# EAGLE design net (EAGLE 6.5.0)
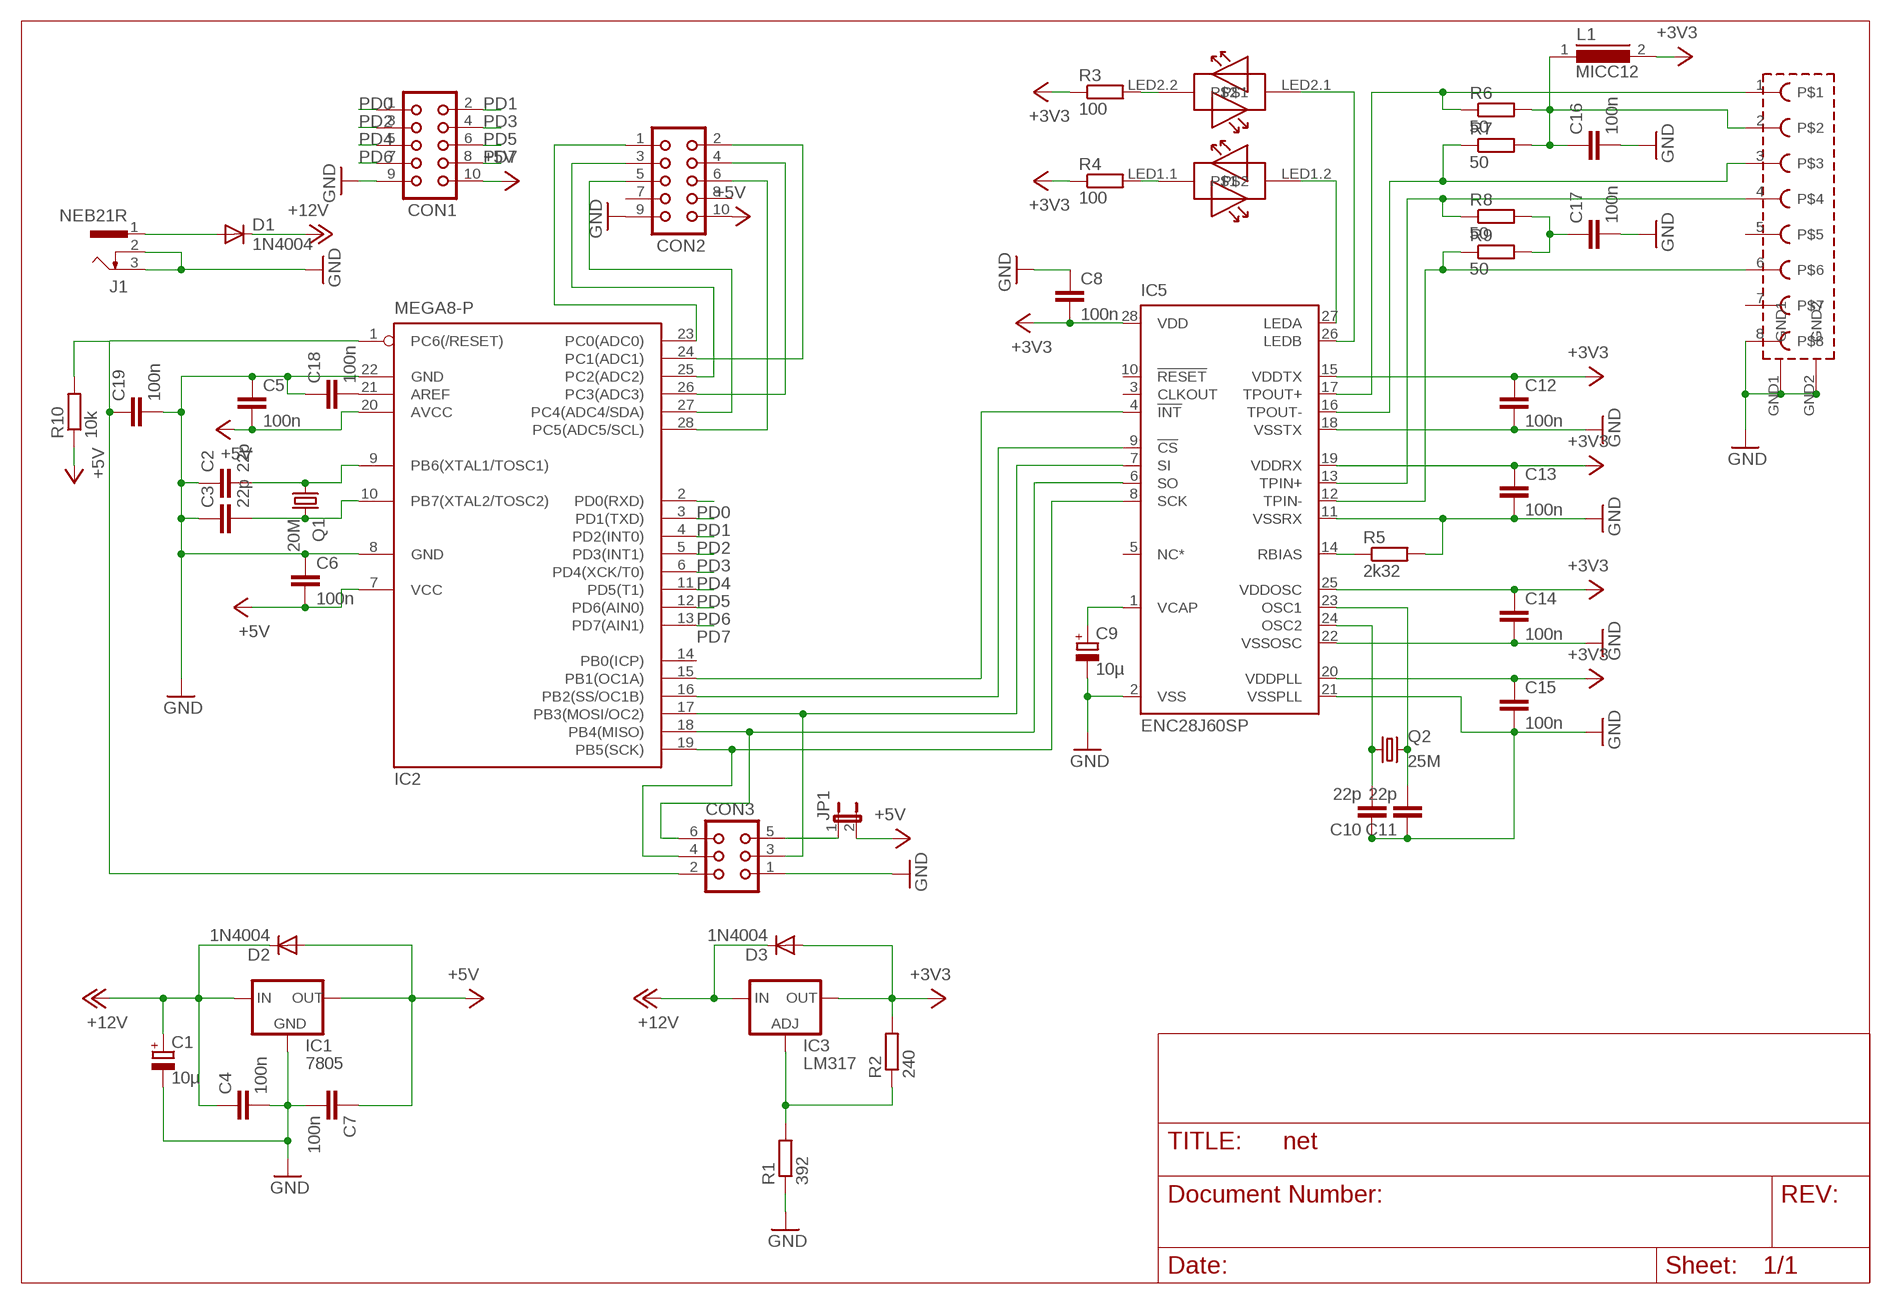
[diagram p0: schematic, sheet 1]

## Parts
C1  10µ  CPOL-EUE2.5-5  [E2,5-5]
C2  22p  C-EU025-025X050  [C025-025X050]
C3  22p  C-EU025-025X050  [C025-025X050]
C4  100n  C-EU025-025X050  [C025-025X050]
C5  100n  C-EU025-025X050  [C025-025X050]
C6  100n  C-EU025-025X050  [C025-025X050]
C7  100n  C-EU025-025X050  [C025-025X050]
C8  100n  C-EU025-025X050  [C025-025X050]
C9  10µ  CPOL-EUE2-4  [E2-4]
C10  22p  C-EU025-025X050  [C025-025X050]
C11  22p  C-EU025-025X050  [C025-025X050]
C12  100n  C-EU025-025X050  [C025-025X050]
C13  100n  C-EU025-025X050  [C025-025X050]
C14  100n  C-EU025-025X050  [C025-025X050]
C15  100n  C-EU025-025X050  [C025-025X050]
C16  100n  C-EU025-025X050  [C025-025X050]
C17  100n  C-EU025-025X050  [C025-025X050]
C18  100n  C-EU025-025X050  [C025-025X050]
C19  100n  C-EU025-025X050  [C025-025X050]
CON1  CON10  [CON10]
CON2  CON10  [CON10]
CON3  CON06  [CON06]
D1  1N4004  [DO41-10]
D2  1N4004  [DO41-10]
D3  1N4004  [DO41-10]
IC1  7805  78XXS  [78XXS]
IC2  MEGA8-P  [DIL28-3]
IC3  LM317  LM317TS  [317TS]
IC5  ENC28J60SP  [DIL28-3]
J1  NEB21R  [NEB21R]
JP1  JP1E  [JP1]
L1  MICC12  [MICC12]
Q1  20M  CRYSTALHC49U-V  [HC49U-V]
Q2  25M  CRYSTALHC49U-V  [HC49U-V]
R1  392  R-EU_0207/10  [0207/10]
R2  240  R-EU_0207/10  [0207/10]
R3  100  R-EU_0207/10  [0207/10]
R4  100  R-EU_0207/10  [0207/10]
R5  2k32  R-EU_0207/10  [0207/10]
R6  50  R-EU_0207/10  [0207/10]
R7  50  R-EU_0207/10  [0207/10]
R8  50  R-EU_0207/10  [0207/10]
R9  50  R-EU_0207/10  [0207/10]
R10  10k  R-EU_0207/10  [0207/10]
U$1  MAGJACK  [MAGJACK]

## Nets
+3V3: C8.2 C12.1 C13.1 C14.1 C15.1 D3.A IC3.2(OUT) IC5.15(VDDTX) IC5.19(VDDRX) IC5.20(VDDPLL) IC5.25(VDDOSC) IC5.28(VDD) L1.2 R2.2 R3.1 R4.1
+5V: C5.2 C6.2 C7.1 CON1.10 CON2.10 D2.A IC1.OUT IC2.7(VCC) IC2.20(AVCC) JP1.2 R10.1
+12V: C1.+ C4.1 D1.C D2.C D3.C IC1.IN IC3.3(IN)
GND: C1.- C2.1 C3.1 C4.2 C5.1 C6.1 C7.2 C8.1 C9.- C10.1 C11.1 C12.2 C13.2 C14.2 C15.2 C16.2 C17.2 C18.1 C19.2 CON1.9 CON2.9 CON3.1 IC1.GND IC2.8(GND) IC2.22(GND) IC5.2(VSS) IC5.11(VSSRX) IC5.18(VSSTX) IC5.21(VSSPLL) IC5.22(VSSOSC) J1.2 J1.3 R1.1 R5.2 U$1.8 U$1.GND1 U$1.GND2
N$1: CON3.5 JP1.1
N$2: CON3.6 IC2.18(PB4(MISO)) IC5.6(SO)
N$3: IC2.16(PB2(SS/OC1B)) IC5.9(!CS)
N$4: IC2.15(PB1(OC1A)) IC5.4(!INT)
N$5: C2.2 IC2.9(PB6(XTAL1/TOSC1)) Q1.1
N$6: C3.2 IC2.10(PB7(XTAL2/TOSC2)) Q1.2
N$7: C9.+ IC5.1(VCAP)
N$8: IC5.14(RBIAS) R5.1
N$10: IC5.17(TPOUT+) R6.1 U$1.1
N$11: R4.2 U$1.LED1.1
N$12: CON3.3 IC2.17(PB3(MOSI/OC2)) IC5.7(SI)
N$13: IC5.16(TPOUT-) R7.1 U$1.3
N$14: C18.2 IC2.21(AREF)
N$15: IC5.13(TPIN+) R8.1 U$1.4
N$16: C10.2 IC5.24(OSC2) Q2.1
N$17: C11.2 IC5.23(OSC1) Q2.2
N$18: IC5.12(TPIN-) R9.1 U$1.6
N$19: C16.1 L1.1 R6.2 R7.2 U$1.2
N$20: C17.1 R8.2 R9.2
N$21: D1.A J1.1
N$23: R3.2 U$1.LED2.2
N$24: IC5.27(LEDA) U$1.LED1.2
N$25: IC5.26(LEDB) U$1.LED2.1
N$26: CON2.1 IC2.23(PC0(ADC0))
N$27: IC3.1(ADJ) R1.2 R2.1
N$28: CON2.2 IC2.24(PC1(ADC1))
N$29: CON2.3 IC2.25(PC2(ADC2))
N$30: CON2.5 IC2.27(PC4(ADC4/SDA))
N$31: CON2.4 IC2.26(PC3(ADC3))
N$32: CON2.6 IC2.28(PC5(ADC5/SCL))
N$34: CON3.4 IC2.19(PB5(SCK)) IC5.8(SCK)
N$37: C19.1 CON3.2 IC2.1(PC6(/RESET)) R10.2
PD0: CON1.1 IC2.2(PD0(RXD))
PD1: CON1.2 IC2.3(PD1(TXD))
PD2: CON1.3 IC2.4(PD2(INT0))
PD3: CON1.4 IC2.5(PD3(INT1))
PD4: CON1.5 IC2.6(PD4(XCK/T0))
PD5: CON1.6 IC2.11(PD5(T1))
PD6: CON1.7 IC2.12(PD6(AIN0))
PD7: CON1.8 IC2.13(PD7(AIN1))
Unconnected: CON2.7 CON2.8 IC2.14(PB0(ICP)) IC5.3(CLKOUT) IC5.5(NC*) IC5.10(!RESET) U$1.5 U$1.7

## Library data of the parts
C1 C9 = rcl:CPOL-EU: POLARIZED CAPACITOR, European symbol
C2 C3 C5 C6 C8 C10-C19 = resistor:C-EU: CAPACITOR, European symbol
C4 C7 = rcl:C-EU: CAPACITOR, European symbol
CON1 CON2 = con-harting:CON10: CONNECTOR; OC_FARNELL: unknown; OC_NEWARK: unknown
CON3 = con-harting:CON06: CONNECTOR; OC_FARNELL: unknown; OC_NEWARK: unknown
D1-D3 = diode:1N4004: DIODE
IC1 = v-reg:78XXS: VOLTAGE REGULATOR
IC2 = atmel:MEGA8-P: MICROCONTROLLER 8 Kbytes FLASH, 1 kbytes SRAM, 512 bytes EEPROM, USART, 4-channel 10 bit ADC, 2-channel 8 bit ADC Pin compatible with Atmega48, ATMega88, ATMega168 Source: avr.lbr; OC_FARNELL: unknown; OC_NEWARK: unknown
IC3 = v-reg:LM317TS: VOLTAGE REGULATOR
IC5 = microchip:ENC28J60: Stand-Alone Ethernet Controller with SPI Interface Source: http://ww1.microchip.com/downloads/en/DeviceDoc/39662c.pdf; MF: MICROCHIP; MPN: ENC28J60/SP; OC_FARNELL: 1084619; OC_NEWARK: 96K3661
J1 = con-lumberg:NEB21R: Netzgeräte-Einbaukupplung abgewinkelte Ausführung mit Öffner Source: http://www.lumberg.com/Produkte/PDFs/NEB21R.pdf; MPN: NEB 21 R; OC_FARNELL: 1217037; OC_NEWARK: 97K6458
JP1 = jumper:JP1E: JUMPER
L1 = inductors:MICC12: INDUCTOR
Q1 Q2 = crystal:CRYSTAL: CRYSTAL; OC_FARNELL: 1666969; OC_NEWARK: unknown
R1-R10 = rcl:R-EU_: RESISTOR, European symbol
U$1 = magjacksmalldrill:MAGJACK

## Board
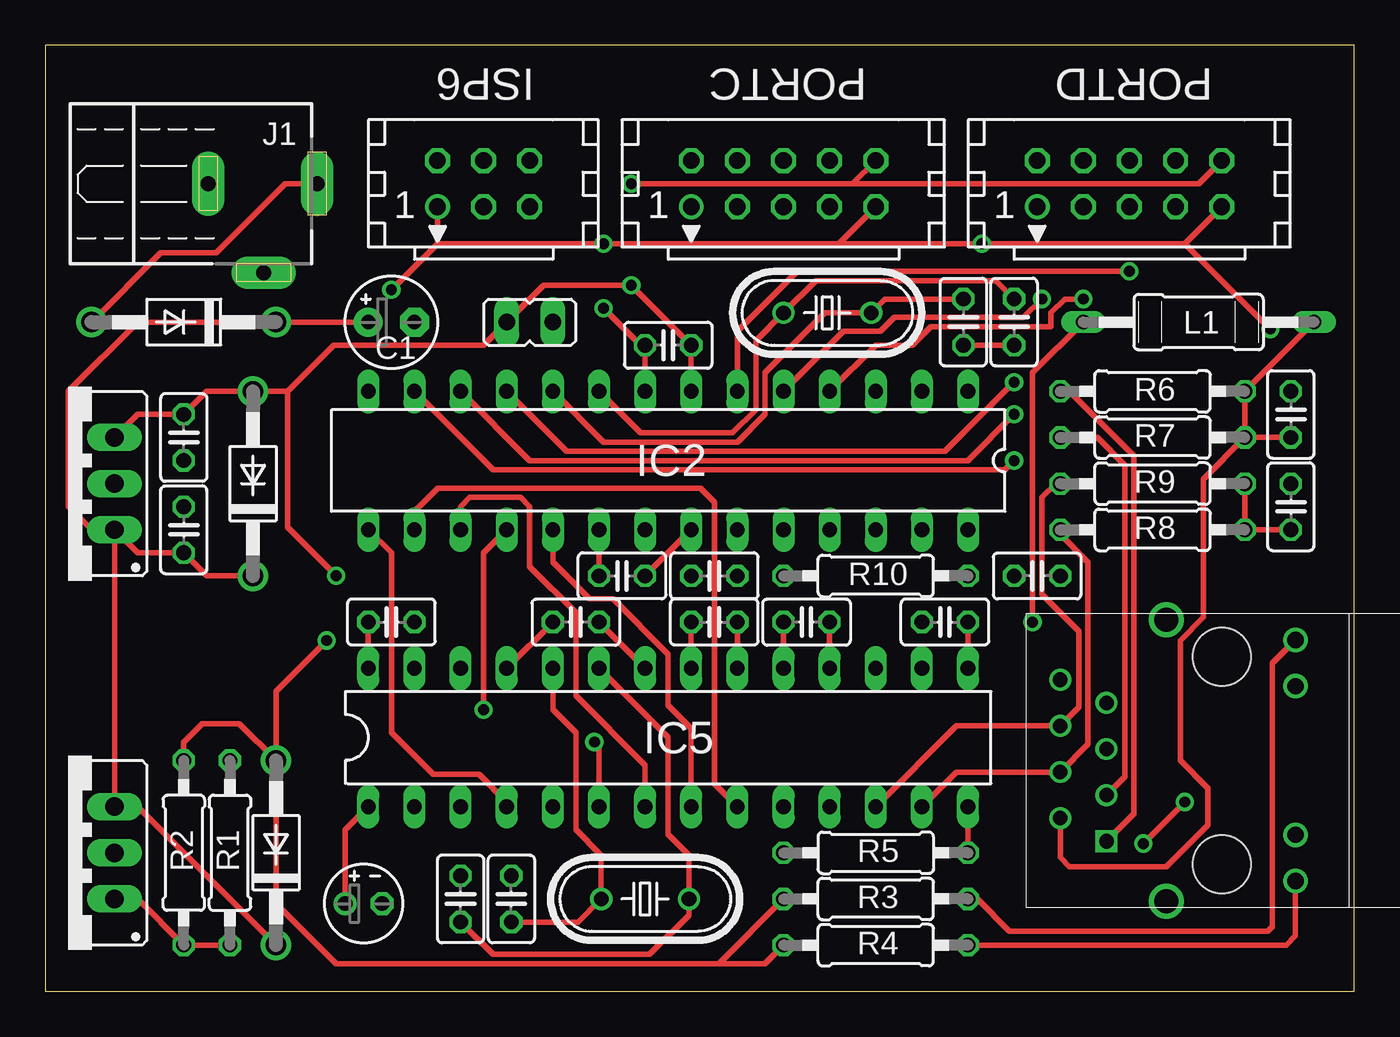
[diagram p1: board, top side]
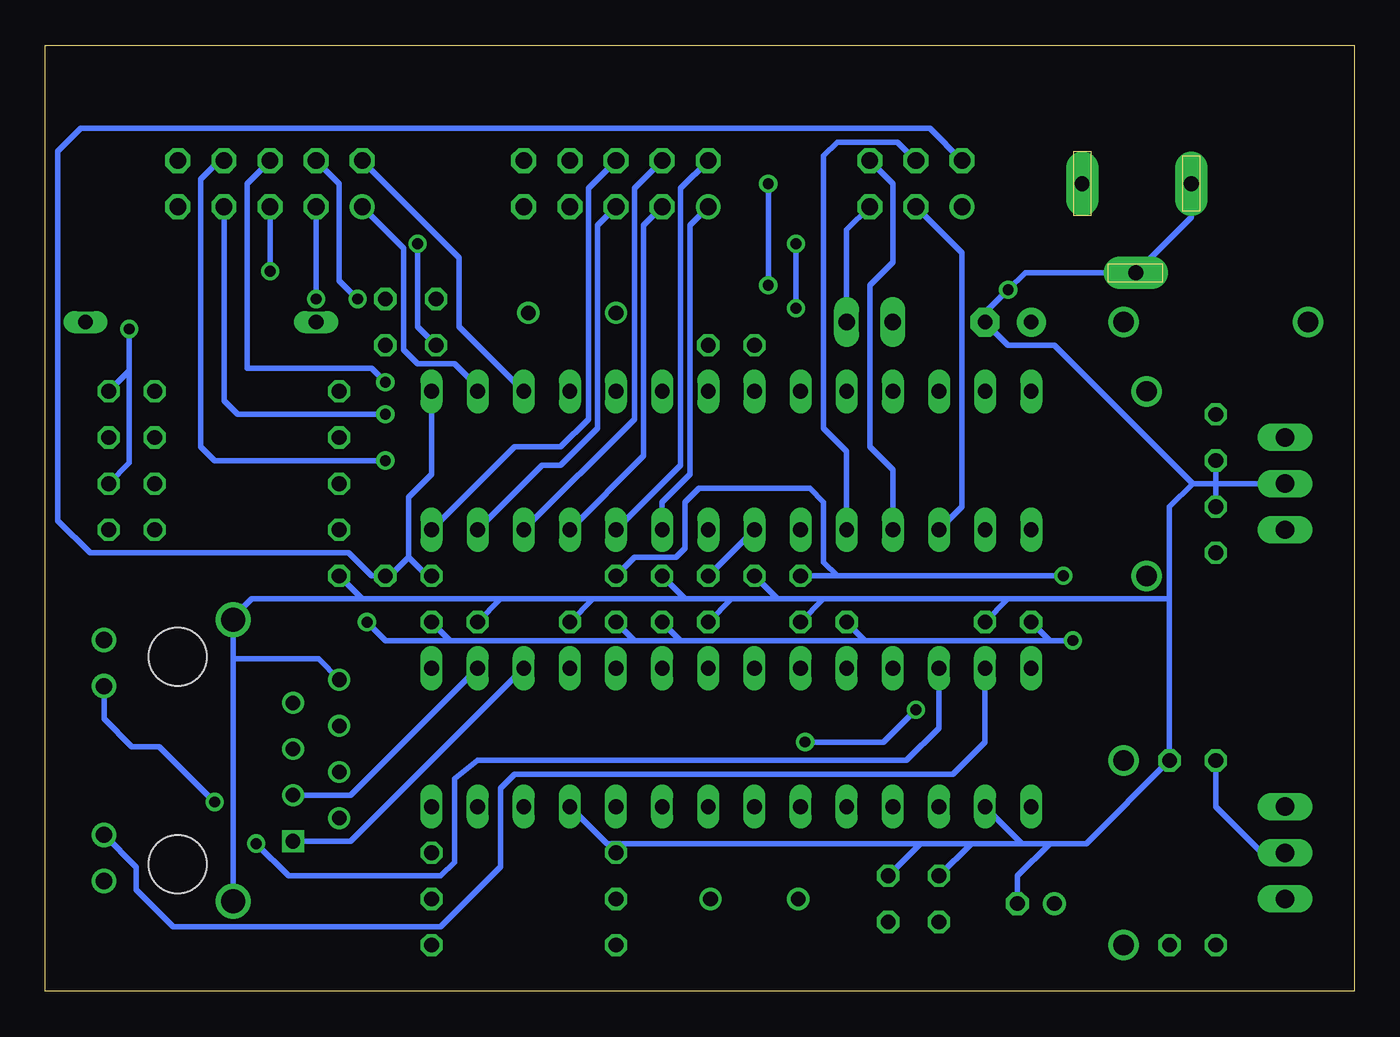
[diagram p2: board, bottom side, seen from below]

Size 72.06 x 52.06 mm. Coordinates in mm from the lower left corner, seen from the top.
Outline: 0,0 72.06,0 72.06,52.06 0,52.06 0,0
Copper layers (1*16): Top 0.035mm / dielectric 1.5mm / Bottom 0.035mm
Design rules "platinensammler_02": minimum track width 0.15mm, minimum drill 0.3mm, track to track 0.15mm, track to pad 0.15mm, pad to pad 0.15mm, via to via 0.15mm, smd to smd 0mil, copper to edge 0.2mm, drill to drill 0.2mm, minimum pad ring 0.2mm, minimum via ring 0.2mm, stop-mask expansion 4mil, vias tented up to drill 0.8mm, thermal gap 0.15mm

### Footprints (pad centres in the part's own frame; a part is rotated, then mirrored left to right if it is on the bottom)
E2,5-5 = drill 0.813 pad 1.6: + -1.27,0 | drill 0.813 pad 1.6 octagon: - 1.27,0
C025-025X050 = drill 0.813 octagon: 1 -1.27,0; 2 1.27,0
E2-4 = drill 0.813 pad 1.27: + -1.016,0 | drill 0.813 pad 1.27 octagon: - 1.016,0
CON10 = drill 0.914: 1 -5.08,-1.27 | drill 0.914 octagon: 2 -5.08,1.27; 3 -2.54,-1.27; 4 -2.54,1.27; 5 0,-1.27; 6 0,1.27; 7 2.54,-1.27; 8 2.54,1.27; 9 5.08,-1.27; 10 5.08,1.27
CON06 = drill 0.914: 1 -2.54,-1.27 | drill 0.914 octagon: 2 -2.54,1.27; 3 0,-1.27; 4 0,1.27; 5 2.54,-1.27; 6 2.54,1.27
DO41-10 = drill 1.118: A 5.08,0; C -5.08,0
78XXS = drill 1.016 long: GND 0,-2.54; IN -2.54,-2.54; OUT 2.54,-2.54
DIL28-3 = drill 0.813 long: 1 -16.51,-3.81; 2 -13.97,-3.81; 3 -11.43,-3.81; 4 -8.89,-3.81; 5 -6.35,-3.81; 6 -3.81,-3.81; 7 -1.27,-3.81; 8 1.27,-3.81; 9 3.81,-3.81; 10 6.35,-3.81; 11 8.89,-3.81; 12 11.43,-3.81; 13 13.97,-3.81; 14 16.51,-3.81; 15 16.51,3.81; 16 13.97,3.81; 17 11.43,3.81; 18 8.89,3.81; 19 6.35,3.81; 20 3.81,3.81; 21 1.27,3.81; 22 -1.27,3.81; 23 -3.81,3.81; 24 -6.35,3.81; 25 -8.89,3.81; 26 -11.43,3.81; 27 -13.97,3.81; 28 -16.51,3.81
317TS = drill 1.016 long: 1 -2.54,-2.54; 2 0,-2.54; 3 2.54,-2.54
NEB21R = drill 0.813 pad 1.778 long: 1 0,7.35; 2 4.9,4.4; 3 0,1.35
JP1 = drill 0.914 long: 1 0,-1.27; 2 0,1.27
MICC12 = drill 0.813 long: 1 -6.35,0; 2 6.35,0
HC49U-V = drill 0.813: 1 -2.413,0; 2 2.413,0
0207/10 = drill 0.813 octagon: 1 -5.08,0; 2 5.08,0
MAGJACK = drill 0.8 square: 1 -4.445,6.35 | drill 0.8: 2 -3.175,8.89; 3 -1.905,6.35; 4 -0.635,8.89; 5 0.635,6.35; 6 1.905,8.89; 7 3.175,6.35; 8 4.445,8.89 | drill 1.3: GND1 -7.747,3.048; GND2 7.747,3.048 | drill 0.9: LED1.1 -6.629,-4.064; LED1.2 -4.089,-4.064; LED2.1 4.089,-4.064; LED2.2 6.629,-4.064 | hole 3.2: -5.715,0; 5.715,0

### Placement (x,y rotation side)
C1  19.05,36.83 0 top
C2  53.34,36.83 90 top
C3  50.55,36.83 90 top
C4  7.62,25.4 90 top
C5  34.29,35.56 0 top
C6  31.75,22.86 180 top
C7  7.62,30.48 270 top
C8  19.05,20.32 180 top
C9  17.53,4.83 0 top
C10  25.65,5.08 270 top
C11  22.86,5.08 270 top
C12  41.91,20.32 0 top
C13  49.53,20.32 180 top
C14  29.21,20.32 0 top
C15  36.83,20.32 180 top
C16  68.58,31.75 90 top
C17  68.58,26.67 90 top
C18  36.83,22.86 180 top
C19  54.61,22.86 0 top
CON1  59.69,44.45 0 top
CON2  40.64,44.45 0 top
CON3  24.13,44.45 0 top
D1  7.62,36.83 180 top
D2  11.43,27.94 90 top
D3  12.7,7.62 90 top
IC1  1.27,27.94 90 top
IC2  34.29,29.21 180 top
IC3  1.27,7.62 90 top
IC5  34.29,13.97 0 top
J1  7.62,44.45 270 top
JP1  26.67,36.83 90 top
L1  63.5,36.83 180 top
Q1  43.05,37.34 0 top
Q2  33.02,5.08 0 top
R1  10.16,7.62 270 top
R2  7.62,7.62 90 top
R3  45.72,5.08 0 top
R4  45.72,2.54 0 top
R5  45.72,7.62 180 top
R6  60.96,33.02 0 top
R7  60.96,30.48 0 top
R8  60.96,25.4 0 top
R9  60.96,27.94 0 top
R10  45.72,22.86 0 top
U$1  64.77,12.7 90 top

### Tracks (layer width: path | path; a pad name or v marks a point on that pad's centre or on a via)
+3V3  (via drill 0.6)
  Top 0.305: C15.1 IC5.20 | C12.1 IC5.19 | C13.1 IC5.15 | R2.2 7.62,13.72 8.64,14.73 10.67,14.73 D3.A | L1.2 54.36,34.04 v54.36,20.32 | R4.1 39.62,1.52 37.08,1.52 | 37.08,1.52 16,1.52 12.7,4.83 D3.A | R3.1 37.08,1.52 | D3.A 12.7,16.51 v15.49,19.3 | IC5.28 C8.2 | C14.1 IC5.25
  Bottom 0.305: IC3.2 5.08,7.62 7.62,10.16 R2.2 | v15.49,19.3 16.76,19.3 | 16.76,19.3 26.92,19.3 | 26.92,19.3 37.08,19.3 | 37.08,19.3 39.62,19.3 | 39.62,19.3 49.78,19.3 | 49.78,19.3 53.34,19.3 v54.36,20.32 | C8.2 16.76,19.3 | C15.1 37.08,19.3 | C12.1 39.62,19.3 | C13.1 49.78,19.3 | C14.1 26.92,19.3
+5V  (via drill 0.6)
  Top 0.305: IC2.7 C5.2 v32.26,38.86 27.43,38.86 JP1.2 24.13,35.56 15.88,35.56 13.34,33.02 | IC1.OUT 5.08,31.75 C7.1 8.89,33.02 D2.A 13.34,33.02 | 13.34,33.02 13.34,25.53 v16,22.86 | CON1.10 63.5,44.45 44.45,44.45 | 44.45,44.45 v32.26,44.45 | CON2.10 44.45,44.45 | IC2.20 C6.2
  Bottom 0.305: v16,22.86 26.92,22.86 28.45,22.86 | 28.45,22.86 C6.2 | v32.26,44.45 v32.26,38.86 | R10.1 39.62,23.88 37.34,23.88 36.83,24.38 36.83,26.92 36.07,27.69 29.97,27.69 29.21,26.92 29.21,23.62 28.45,22.86
+12V
  Top 0.305: IC1.IN 2.54,25.4 1.27,26.67 1.27,33.02 5.08,36.83 D1.C C1.+ | IC1.IN 5.08,24.13 C4.1 8.89,22.86 D2.C | IC1.IN IC3.3 5.08,10.16 D3.C
GND  (via drill 0.6)
  Top 0.305: IC5.21 C15.2 | IC5.18 C12.2 | C5.1 IC2.8 33.02,35.31 v30.73,37.59 | IC5.22 C14.2 | CON3.1 21.59,41.15 | 21.59,41.15 v19.05,38.61 | CON2.9 43.69,41.15 | 43.69,41.15 v30.73,41.15 21.59,41.15 | CON1.9 62.74,41.15 | 62.74,41.15 v51.56,41.15 43.69,41.15 | C3.1 C2.1 | 62.74,41.15 v67.44,36.45 | IC2.22 C6.1
  Bottom 0.305: IC1.GND 7.62,27.94 | C7.2 7.62,27.94 | C4.2 7.62,27.94 | U$1.GND1 61.72,18.29 | 61.72,18.29 U$1.GND2 61.72,20.57 60.71,21.59 54.61,21.59 | U$1.8 57.02,18.29 61.72,18.29 | 18.29,8.13 16.76,8.13 | 16.76,8.13 14.73,8.13 R1.1 10.16,21.59 | C11.1 21.08,8.13 | 21.08,8.13 18.29,8.13 | C10.1 23.88,8.13 | 23.88,8.13 21.08,8.13 | R5.2 40.13,8.13 | 40.13,8.13 23.88,8.13 | IC5.2 18.29,8.13 | IC5.11 41.15,8.13 40.13,8.13 | 7.62,27.94 8.89,27.94 | 8.89,27.94 10.16,26.67 10.16,21.59 | C13.2 46.99,21.59 | 46.99,21.59 41.91,21.59 | 41.91,21.59 36.83,21.59 | 34.29,21.59 31.75,21.59 | 29.21,21.59 19.05,21.59 | 19.05,21.59 10.16,21.59 | C8.1 19.05,21.59 | C15.2 34.29,21.59 | C12.2 41.91,21.59 | C16.2 67.44,34.16 | C17.2 67.44,29.08 67.44,34.16 | 54.61,21.59 46.99,21.59 | 67.44,34.16 v67.44,36.45 | 8.89,27.94 16.51,35.56 19.05,35.56 C1.- 20.32,37.34 v19.05,38.61 18.11,39.55 J1.2 8.97,42.6 J1.3 | v30.73,37.59 v30.73,41.15 | C3.1 51.56,36.58 v51.56,41.15 | C14.2 29.21,21.59 | C6.1 31.75,21.59 | 31.75,21.59 29.21,21.59 | C18.1 36.83,21.59 | 36.83,21.59 34.29,21.59 | C19.2 54.61,21.59 | C9.- 18.54,6.35 16.76,8.13
N$1
  Bottom 0.305: CON3.5 27.94,41.91 JP1.1
N$2  (via drill 0.6)
  Top 0.305: IC5.6 30.48,13.46 v30.23,13.72 | v24.13,15.49 24.13,24.13 IC2.18
  Bottom 0.305: v30.23,13.72 25.91,13.72 v24.13,15.49 | CON3.6 25.4,44.45 25.4,40.13 26.67,38.86 26.67,29.97 25.4,28.7 IC2.18
N$3
  Top 0.305: IC5.9 36.83,11.43 36.83,26.92 36.07,27.69 21.59,27.69 20.32,26.42 IC2.16
N$4
  Top 0.305: IC2.15 19.05,24.13 19.05,14.22 21.34,11.94 23.88,11.94 25.4,10.41 IC5.4
N$5
  Top 0.305: IC2.9 32.77,30.73 37.85,30.73 39.12,32 39.12,35.81 Q1.1 42.42,39.12 52.32,39.12 C2.2
N$6
  Top 0.305: IC2.10 30.73,30.23 38.1,30.23 39.62,31.75 39.62,34.04 42.93,37.34 Q1.2 46.23,38.1 C3.2
N$7
  Top 0.305: IC5.1 16.51,8.89 C9.+
N$8
  Top 0.305: IC5.14 R5.1
N$10
  Top 0.305: R6.1 56.39,33.02 59.94,29.46 59.94,9.78 U$1.1
  Bottom 0.305: IC5.17 55.24,8.26 U$1.1
N$11
  Top 0.305: U$1.LED1.1 68.83,3.05 68.33,2.54 R4.2
N$12
  Top 0.305: IC5.7 33.02,12.45 29.21,16.26 29.21,20.83 26.67,23.37 26.67,26.67 26.16,27.18 23.37,27.18 22.86,26.67 IC2.17
  Bottom 0.305: CON3.3 21.59,40.64 21.59,26.67 IC2.17
N$13
  Top 0.305: R7.1 57.91,30.48 59.44,28.96 59.44,11.81 U$1.3
  Bottom 0.305: IC5.16 55.24,10.79 U$1.3
N$14
  Bottom 0.305: IC2.21 C18.2
N$15
  Top 0.305: IC5.13 50.16,12.06 U$1.4 57.4,13.59 57.4,23.62 55.88,25.15 R8.1
N$16
  Top 0.305: C10.2 29.34,3.81 Q2.1 30.61,7.49 29.21,8.89 29.21,14.22 27.94,15.49 IC5.24
N$17
  Top 0.305: IC5.23 34.29,13.97 34.29,8.64 35.43,7.49 Q2.2 35.43,4.19 33.27,2.03 24.64,2.03 C11.2
N$18
  Top 0.305: IC5.12 50.16,14.61 U$1.6 56.9,15.62 56.9,19.81 54.86,21.84 54.86,27.18 55.63,27.94 R9.1
N$19
  Top 0.305: R7.2 R6.2 L1.1 | R7.2 C16.1 | R7.2 63.75,28.19 63.75,20.57 62.48,19.3 62.48,12.7 64.01,11.18 64.01,9.14 61.72,6.86 56.39,6.86 55.88,7.37 U$1.2
N$20
  Top 0.305: R9.2 R8.2 C17.1
N$21
  Top 0.305: J1.1 13.21,44.45 9.4,40.64 6.35,40.64 D1.A
N$23
  Top 0.305: U$1.LED2.2 67.56,18.06 67.56,3.56 67.31,3.3 53.09,3.3 51.31,5.08 R3.2
N$24
  Bottom 0.305: IC5.27 20.32,13.72 22.1,11.94 46.23,11.94 46.99,11.18 46.99,6.86 50.29,3.56 65.02,3.56 67.06,5.59 67.06,6.83 U$1.LED1.2
N$25  (via drill 0.6)
  Top 0.305: v60.45,8.13 v62.74,10.41
  Bottom 0.305: IC5.26 22.86,14.48 24.64,12.7 48.26,12.7 49.53,11.68 49.53,7.11 50.29,6.35 58.67,6.35 v60.45,8.13 | v62.74,10.41 65.79,13.46 67.31,13.46 68.83,14.99 U$1.LED2.1
N$26
  Bottom 0.305: CON2.1 36.58,42.16 36.58,28.45 38.1,26.92 IC2.23
N$27
  Top 0.305: IC3.1 5.08,5.08 R2.1 R1.2
N$28
  Bottom 0.305: CON2.2 37.08,44.2 37.08,28.96 IC2.24
N$29
  Bottom 0.305: CON2.3 39.12,42.16 39.12,29.46 IC2.25
N$30
  Bottom 0.305: CON2.5 41.66,42.16 41.66,30.99 43.69,28.96 44.7,28.96 IC2.27
N$31
  Bottom 0.305: CON2.4 39.62,44.2 39.62,31.5 IC2.26
N$32
  Bottom 0.305: CON2.6 42.16,44.2 42.16,31.5 43.69,29.97 46.23,29.97 IC2.28
N$34
  Top 0.305: IC5.8 35.56,14.48 34.29,15.75 34.29,18.54 31.24,21.59 29.97,21.59 27.94,23.62 IC2.19
  Bottom 0.305: CON3.4 25.15,46.74 28.45,46.74 29.21,45.97 29.21,30.99 27.94,29.72 IC2.19
N$37
  Bottom 0.305: IC2.1 50.8,28.45 52.07,27.18 52.07,23.88 | CON3.2 23.37,47.5 70.1,47.5 71.37,46.23 71.37,25.91 69.6,24.13 55.37,24.13 54.1,22.86 C19.1 53.09,22.86 52.07,23.88 | 52.07,23.88 51.05,22.86 R10.2
PD0
  Bottom 0.305: IC2.2 48.26,33.27 49.53,34.54 51.56,34.54 52.32,35.31 52.32,40.89 CON1.1
PD1
  Bottom 0.305: IC2.3 49.28,36.58 49.28,40.39 CON1.2
PD2  (via drill 0.6)
  Top 0.305: IC2.4 45.72,35.56 47.75,35.56 48.77,36.58 55.37,36.58 55.37,37.34 56.13,38.1 v57.15,38.1
  Bottom 0.305: v57.15,38.1 CON1.3
PD3  (via drill 0.6)
  Top 0.305: IC2.5 43.94,36.32 45.97,36.32 46.74,37.08 53.85,37.08 v54.86,38.1
  Bottom 0.305: CON1.4 55.88,44.45 55.88,39.12 v54.86,38.1
PD4  (via drill 0.6)
  Top 0.305: IC2.6 38.1,36.32 41.4,39.62 v59.69,39.62
  Bottom 0.305: v59.69,39.62 CON1.5
PD5  (via drill 0.6)
  Top 0.305: IC2.11 28.7,29.72 49.53,29.72 v53.34,33.53
  Bottom 0.305: v53.34,33.53 54.1,34.29 60.96,34.29 60.96,44.45 CON1.6
PD6  (via drill 0.6)
  Top 0.305: IC2.12 26.67,29.21 50.8,29.21 v53.34,31.75
  Bottom 0.305: v53.34,31.75 61.47,31.75 62.23,32.51 CON1.7
PD7  (via drill 0.6)
  Top 0.305: IC2.13 24.64,28.7 52.83,28.7 v53.34,29.21
  Bottom 0.305: v53.34,29.21 62.74,29.21 63.5,29.97 63.5,44.7 62.48,45.72 CON1.8

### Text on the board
tNames: ISP6 | PORTC | PORTD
